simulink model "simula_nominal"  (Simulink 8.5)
settings: Solver=ode45  StartTime=0.0  StopTime=tf  RelTol=1e-3
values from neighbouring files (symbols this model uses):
  denK = conv([1/3 1],[1 0.01])    [princi_JL_incerto_sem_prefilt_com_limit_ctrle.m]
  knom = r*kT/Ra/Jeq    [princi_JL_incerto_sem_prefilt_com_limit_ctrle.m]
  numK = 3.5*0.1*[1 0.1]    [princi_JL_incerto_sem_prefilt_com_limit_ctrle.m]
  pnom = feq/Jeq    [princi_JL_incerto_sem_prefilt_com_limit_ctrle.m]
undefined symbols (not defined in the file or in its folder): denF, numF, w0

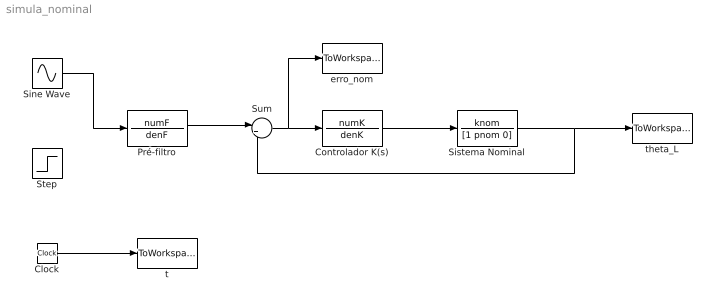
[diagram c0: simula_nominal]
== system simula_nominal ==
  Clock : Clock
  Controlador K(s) : TransferFcn  Numerator=numK  Denominator=denK
  Pré-filtro : TransferFcn  Numerator=numF  Denominator=denF
  Sine Wave : Sin  Frequency=w0  SampleTime=0
  Sistema Nominal : TransferFcn  Numerator=knom  Denominator=[1 pnom 0]
  Step : Step  Time=0  SampleTime=0
  Sum : Sum  Inputs=|+-
  erro_nom : ToWorkspace  VariableName=erro_nom  SampleTime=-1
  t : ToWorkspace  VariableName=t  SampleTime=-1
  theta_L : ToWorkspace  VariableName=theta_L_nom  SampleTime=-1
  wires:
  Sum/1 -> erro_nom/1, Controlador K(s)/1
  Pré-filtro/1 -> Sum/1
  Clock/1 -> t/1
  Controlador K(s)/1 -> Sistema Nominal/1
  Sistema Nominal/1 -> Sum/2, theta_L/1
  Sine Wave/1 -> Pré-filtro/1
